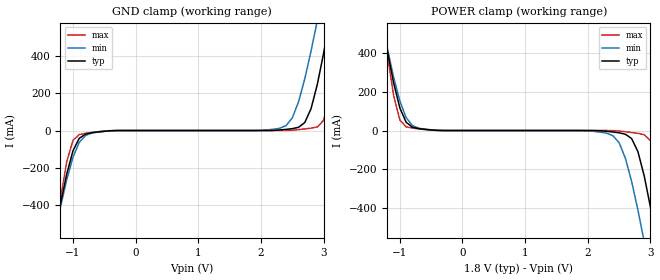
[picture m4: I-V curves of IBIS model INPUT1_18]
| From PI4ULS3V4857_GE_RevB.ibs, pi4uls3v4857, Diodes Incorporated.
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[Model] INPUT1_18
Model_type Input
Vinl = 0.36V
Vinh = 1.44V
| variable   typ   min   max
C_comp   5.931pF   5.877pF   5.999pF
[Voltage Range]   1.8V   1.6V   2.0V
[GND Clamp Reference]   0.000V   0.000V   0.000V
[POWER Clamp Reference]   1.8V   1.6V   2.0V
[temperature range]   40   85   -40
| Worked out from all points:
|   GND clamp passes 1 mA (typ) near -0.38 V on its own axis
|   POWER clamp passes 1 mA (typ) near -0.41 V on its own axis
[GND Clamp]
| Voltage   I(typ)   I(min)   I(max)
-1.8V     -1.62A     -1.49A     -1.99A
-1.3V     -580mA     -574mA     -609mA
-1.1V     -234mA     -264mA     -168mA
-900mV    -41.8mA    -63.2mA    -21.6mA
-400mV    -1.24mA    -1.75mA    -426uA
2.4V      6.14mA     26mA       260uA
2.7V      42.8mA     277mA      8.62mA
2.9V      247mA      589mA      19.3mA
3V        413mA      762mA      54.6mA
3.1V      599mA      940mA      182mA
3.3V      1A         1.31A      644mA
3.6V      1.64A      1.88A      1.49A
[POWER Clamp]   |Note: Vtable = Vcc - Voutput
| Voltage   I(typ)   I(min)   I(max)
-1.8V     1.64A      1.5A       2.08A
-1.3V     599mA      589mA      644mA
-1.1V     247mA      277mA      182mA
-1V       117mA      153mA      54.6mA
-900mV    42.8mA     67.2mA     19.3mA
-500mV    3.02mA     3.61mA     1.93mA
2.4V      -7.57mA    -26.5mA    -426uA
2.7V      -41.8mA    -264mA     -10.4mA
2.9V      -234mA     -574mA     -21.6mA
3.1V      -580mA     -927mA     -168mA
3.3V      -980mA     -1.3A      -609mA
3.6V      -1.62A     -1.88A     -1.42A
